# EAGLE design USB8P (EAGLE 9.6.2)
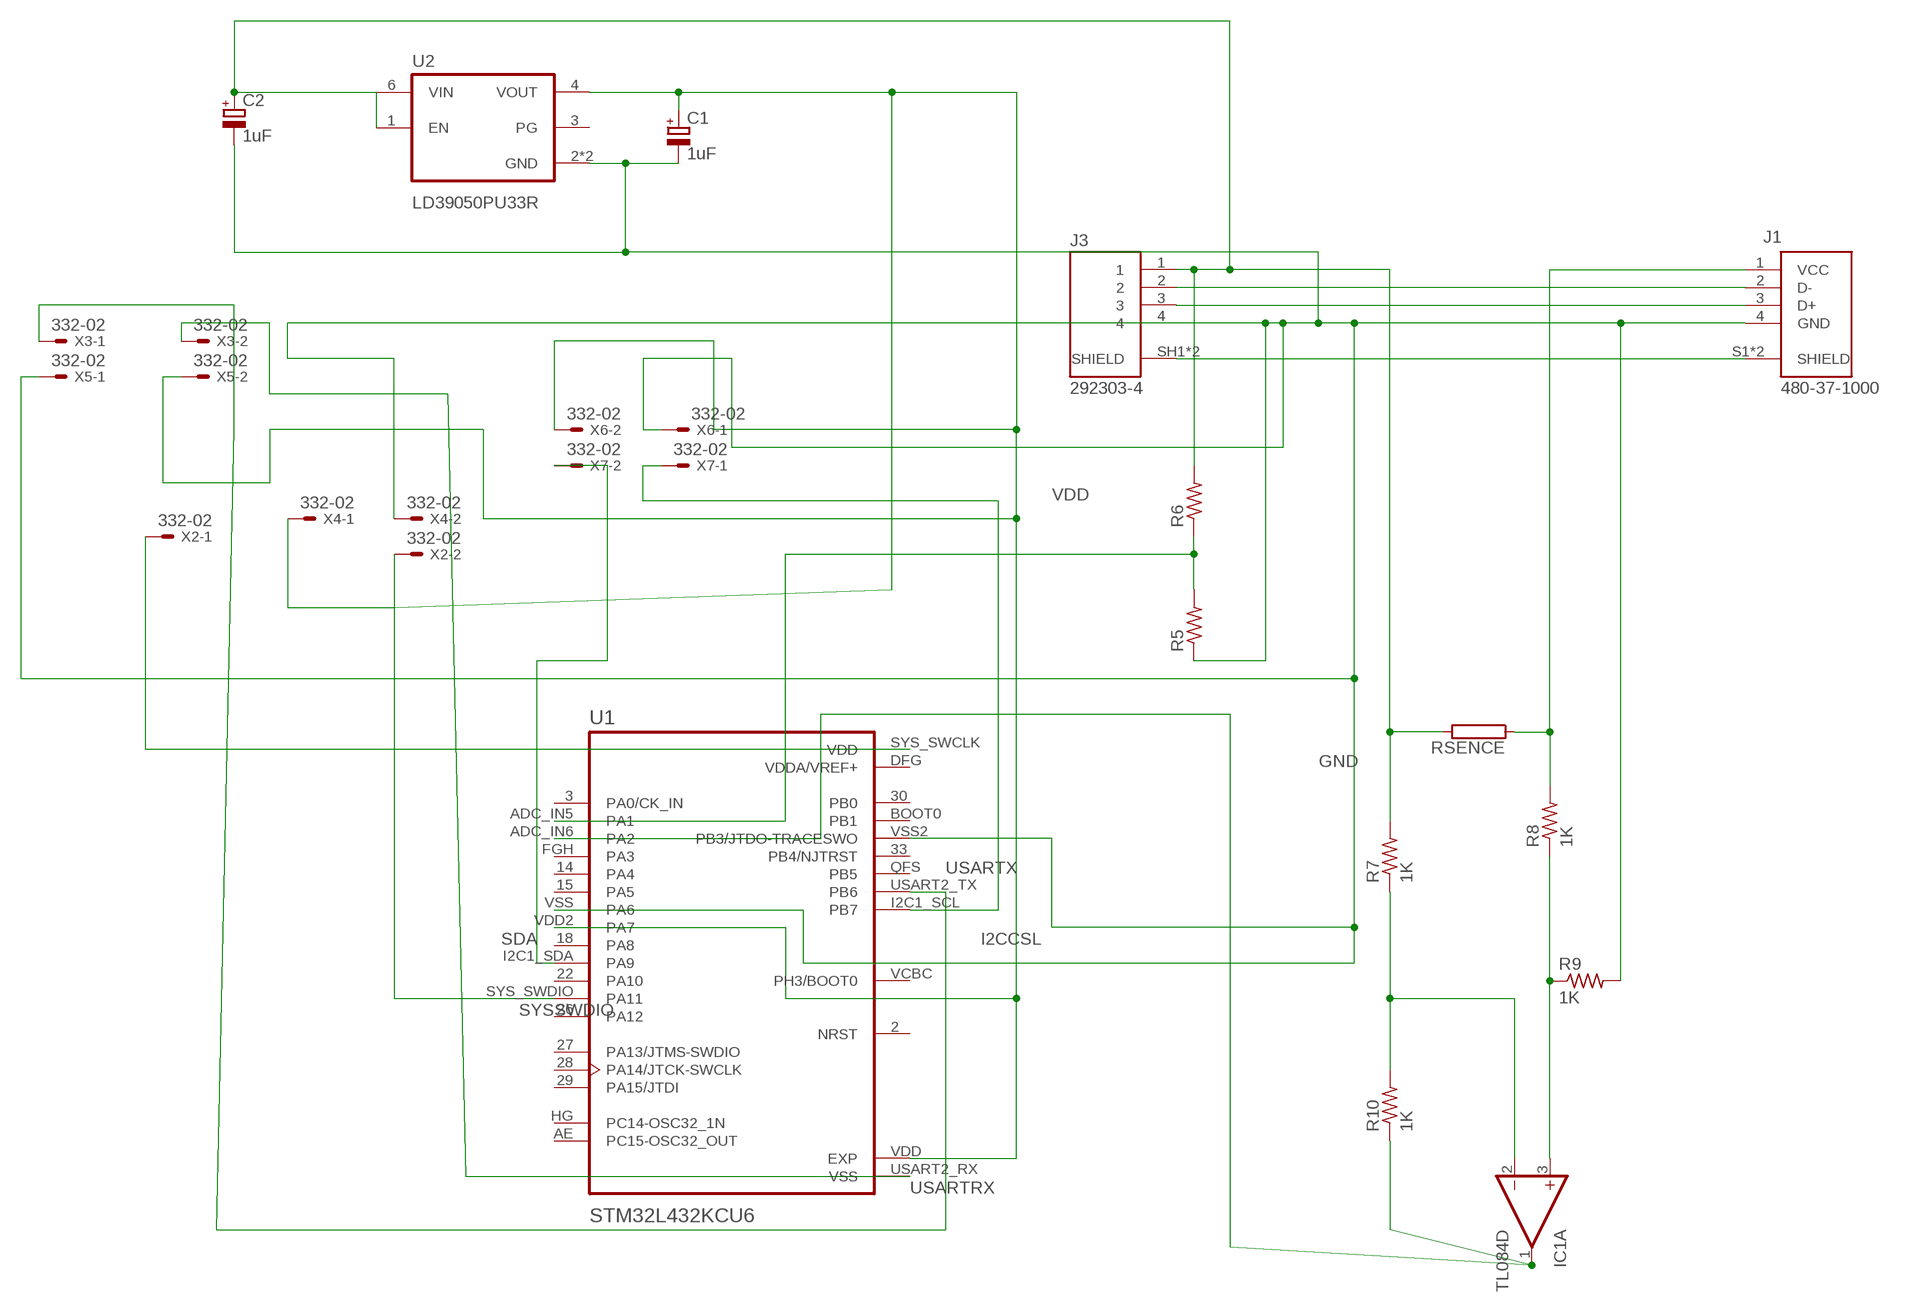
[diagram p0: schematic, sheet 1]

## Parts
C1  1uF  CPOL-EUE1.8-4  [E1,8-4]
C2  1uF  CPOL-EUE1.8-4  [E1,8-4]
IC1  TL084D  [SO14]
J1  480-37-1000  [MOLEX_480-37-1000]
J3  292303-4  [TE_292303-4]
R5  R-US_R1206  [R1206]
R6  R-US_R1206  [R1206]
R7  1K  R-US_R1206  [R1206]
R8  1K  R-US_R1206  [R1206]
R9  1K  R-US_R1206  [R1206]
R10  1K  R-US_R1206  [R1206]
RSENCE  RHPS58  [HPS58]
U1  STM32L432KCU6  [QFN50P500X500X60-33N]
U2  LD39050PU33R  [SON95P300X300X100-7N]
X2  332-02  [332-02]
X3  332-02  [332-02]
X4  332-02  [332-02]
X5  332-02  [332-02]
X6  332-02  [332-02]
X7  332-02  [332-02]

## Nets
GND: C1.- C2.- J1.4(GND) J3.4 R5.1 R9.2 U1.VSS2(PB3/JTDO-TRACESWO) U1.VSS(PA6) U2.2(GND) U2.7(GND) X4.2 X5.1 X6.1
I2CCSL: U1.I2C1_SCL(PB7) X7.1
N$1: IC1.2(A:-IN) R7.1 R10.2
N$2: IC1.3(A:+IN) R8.1 R9.1
N$3: IC1.1(A:OUT) R10.1 U1.ADC_IN6(PA2)
N$4: C2.+ J3.1 R6.2 R7.2 RSENCE.2 U2.1(EN) U2.6(VIN)
N$6: J1.2(D-) J3.2
N$7: J1.3(D+) J3.3
N$9: J1.S1(SHIELD) J1.S2(SHIELD) J3.SH1(SHIELD) J3.SH2(SHIELD)
N$10: R5.2 R6.1 U1.ADC_IN5(PA1)
N$12: U1.SYS_SWCLK(VDD) X2.1
SDA: U1.I2C1_SDA(PA9) X7.2
SYSSWDIO: U1.SYS_SWDIO(PA11) X2.2
USARTRX: U1.USART2_RX(VSS) X3.2
USARTX: U1.USART2_TX(PB6) X3.1
VCC: J1.1(VCC) R8.2 RSENCE.1
VDD: C1.+ U1.VDD2(PA7) U1.VDD(EXP) U2.4(VOUT) X4.1 X5.2 X6.2
Unconnected: IC1.5(B:+IN) IC1.6(B:-IN) IC1.7(B:OUT) IC1.8(C:OUT) IC1.9(C:-IN) IC1.10(C:+IN) IC1.12(D:+IN) IC1.13(D:-IN) IC1.14(D:OUT) U1.2(NRST) U1.3(PA0/CK_IN) U1.14(PA4) U1.15(PA5) U1.18(PA8) U1.22(PA10) U1.26(PA12) U1.27(PA13/JTMS-SWDIO) U1.28(PA14/JTCK-SWCLK) U1.29(PA15/JTDI) U1.30(PB0) U1.33(PB4/NJTRST) U1.AE(PC15-OSC32_OUT) U1.BOOT0(PB1) U1.FGH(PA3) U1.HG(PC14-OSC32_1N) U1.QFS(PB5) U1.VCBC(PH3/BOOT0) U2.3(PG)

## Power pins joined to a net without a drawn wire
GND: IC1.11(P:V-)
VCC: IC1.4(P:V+)
VDDA/VREF+: U1.DFG(VDDA/VREF+)

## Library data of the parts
C1 C2 = rcl:CPOL-EU: POLARIZED CAPACITOR, European symbol; SPICEPREFIX: C
IC1 = linear:TL084: OP AMP
J1 = 480-37-1000:480-37-1000: USB-A (USB TYPE-A) USB 2.0 Plug Connector 4 Position Surface Mount, Right Angle; Through Hole; AVAILABILITY: Unavailable; DESCRIPTION: USB-A (USB TYPE-A) USB 2.0 Plug Connector 4 Position Surface Mount, Right Angle; Through Hole; MF: Molex; MP: 480-37-1000; PACKAGE: FakePackage u; PRICE: None
J3 = 292303-4:292303-4: CONN USB TYPE A R/A PCB Check prices; AVAILABILITY: Good; COMMENT: 292303-4; DESCRIPTION: Conn; Data; USB; Recept; 2.0; 4 Pos; 1 Port; Rt Angle; A Ser; Tin over Copper; EU_ROHS_COMPLIANCE: Compliant; MF: TE Connectivity; MP: 292303-4; PACKAGE: None; PRICE: None; PURCHASE-URL: https://pricing.snapeda.com/search/part/292303-4/?ref=eda
R5-R10 = rcl:R-US_: RESISTOR, American symbol; SPICEPREFIX: R
RSENCE = resistor-power:R: Power Resitor; OC_FARNELL: unknown; OC_NEWARK: unknown
U1 = STM32G030K6:STM32L432KCU6: None Check prices; AVAILABILITY: Good; DESCRIPTION: ARM® Cortex®-M4 STM32L4 Microcontroller IC 32-Bit 80MHz 256KB (256K x 8) FLASH 32-UFQFPN (5x5); MF: STMicroelectronics; MP: STM32L432KCU6; PACKAGE: UFQFN-32 STMicroelectronics; PRICE: None; PURCHASE-URL: https://pricing.snapeda.com/search/part/STM32L432KCU6/?ref=eda
U2 = LD39050PU33R:LD39050PU33R: LD39050 Series 500 mA 3.3 V Fixed Low Noise LDO Voltage Regulator - DFN-6 Check prices; AVAILABILITY: Good; DESCRIPTION: Linear Voltage Regulator IC Positive Fixed 1 Output 500mA 6-DFN (3x3); MF: STMicroelectronics; MP: LD39050PU33R; PACKAGE: DFN-6 STMicroelectronics; PRICE: None; PURCHASE-URL: https://pricing.snapeda.com/search/part/LD39050PU33R/?ref=eda
X2-X7 = con-garry:332-02: 2 Pin - 2mm Dual Row

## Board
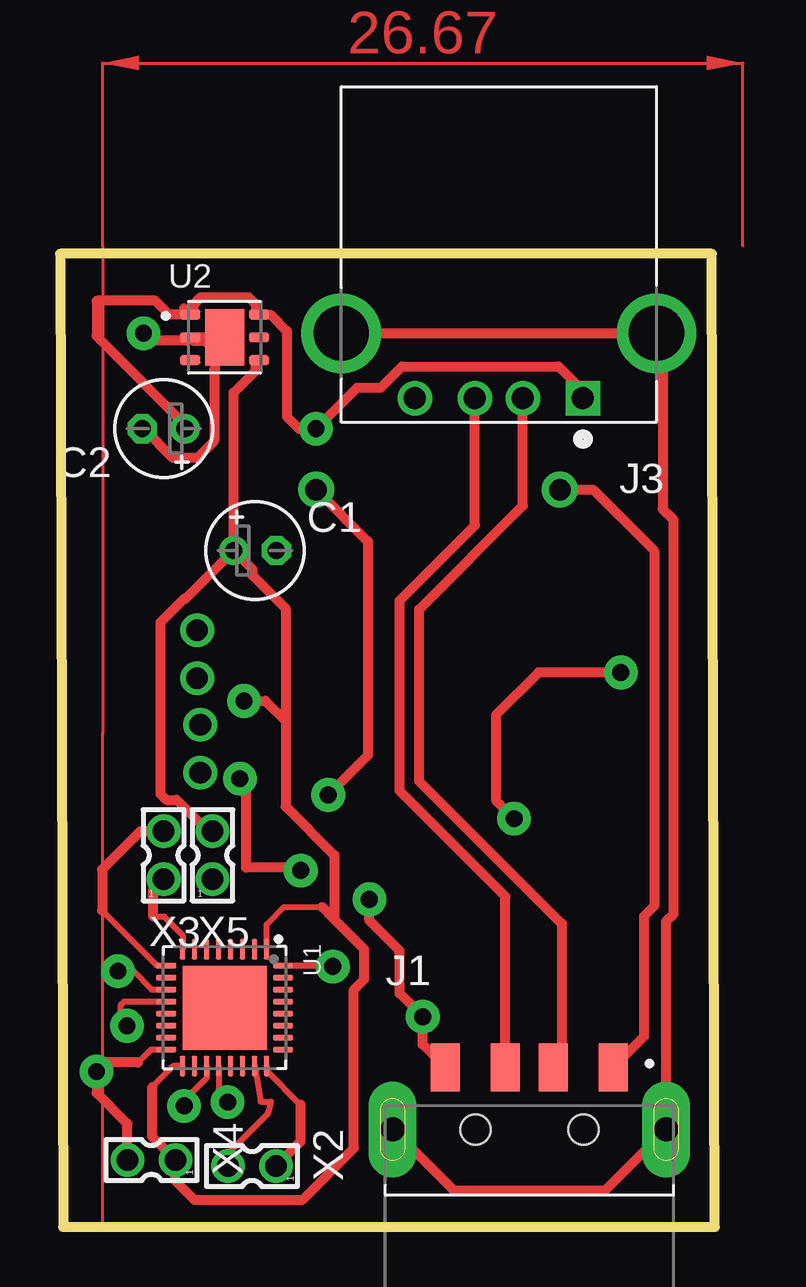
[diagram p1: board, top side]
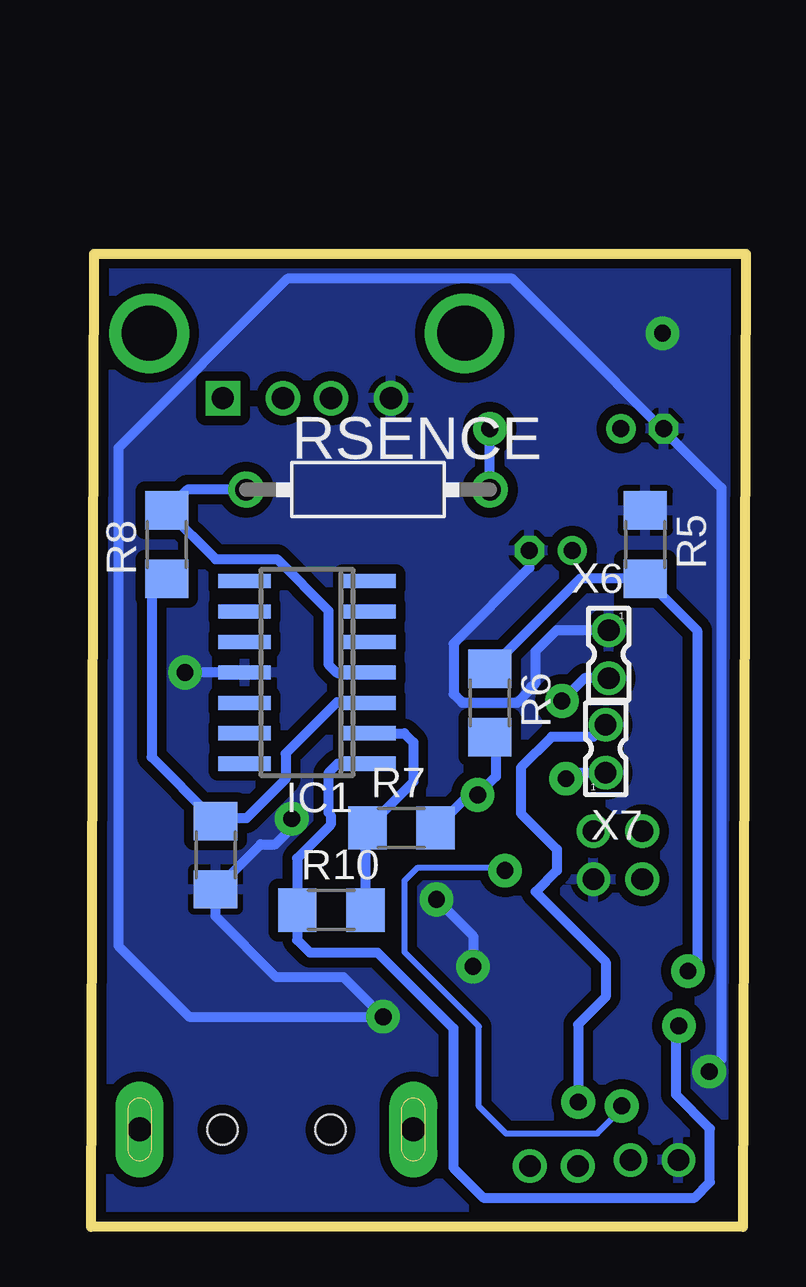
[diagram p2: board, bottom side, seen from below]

Size 27.29 x 40.56 mm. Coordinates in mm from the lower left corner, seen from the top.
Outline: 0.13,0 27.29,0 27.16,40.56 0,40.56 0.13,0
Copper layers (1*16): Top 0.035mm / dielectric 1.5mm / Bottom 0.035mm
Design rules "default *": minimum track width 16mil, minimum drill 0.35mm, track to track 16mil, track to pad 16mil, pad to pad 16mil, via to via 16mil, smd to smd 16mil, copper to edge 16mil, drill to drill 6mil, minimum pad ring 10mil, minimum via ring 8mil, stop-mask expansion 4mil, vias tented up to drill 0mil, thermal gap 10mil

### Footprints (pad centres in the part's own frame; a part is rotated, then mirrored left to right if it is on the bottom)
E1,8-4 = drill 0.711 pad 1.168: + -0.889,0 | drill 0.711 pad 1.168 octagon: - 0.889,0
SO14 = smd 0.6 x 2.2: 1 -3.81,-2.6; 2 -2.54,-2.6; 3 -1.27,-2.6; 4 0,-2.6; 5 1.27,-2.6; 6 2.54,-2.6; 7 3.81,-2.6; 8 3.81,2.6; 9 2.54,2.6; 10 1.27,2.6; 11 0,2.6; 12 -1.27,2.6; 13 -2.54,2.6; 14 -3.81,2.6
MOLEX_480-37-1000 = smd 1.2 x 2: 1 3.5,2.6; 2 1,2.6; 3 -1,2.6; 4 -3.5,2.6 | drill 1 pad 2 long: S1 -5.7,0; S2 5.7,0 | hole 1.25: -2.25,0; 2.25,0
TE_292303-4 = drill 0.92 square: 1 -3.5,0 | drill 0.92: 2 -1,0; 3 1,0; 4 3.5,0 | drill 2.3: SH1 -6.57,-2.71; SH2 6.57,-2.71
R1206 = smd 1.6 x 1.803: 1 -1.422,0; 2 1.422,0
HPS58 = drill 0.9 pad 1.5: 1 -5.08,0; 2 5.08,0
QFN50P500X500X60-33N = smd 0.86 x 0.25: 2 -2.435,1.25; 3 -2.435,0.75; 18 2.435,-1.25; 22 2.435,0.75; AE -2.435,-0.75; HG 2.435,0.25; I2C1_SCL 2.435,-0.75; I2C1_SDA 2.435,-0.25; NRST -2.435,0.25; QFS -2.435,-1.25; SYS_SWCLK 2.435,1.75; SYS_SWDIO 2.435,1.25; USART2_TX -2.435,-1.75; VDD -2.435,1.75; VDD2 2.435,-1.75; VDDA -2.435,-0.25 | smd 0.25 x 0.86: 14 0.75,-2.435; 15 1.25,-2.435; 26 1.25,2.435; 27 0.75,2.435; 28 0.25,2.435; 29 -0.25,2.435; 30 -0.75,2.435; ADC_IN5 -0.75,-2.435; ADC_IN6 -0.25,-2.435; BOOT0 -1.25,2.435; DFG -1.25,-2.435; FGH 0.25,-2.435; USART2_RX -1.75,-2.435; VCBC 1.75,2.435; VSS 1.75,-2.435; VSS2 -1.75,2.435 | smd 3.5 x 3.5: 33 0,0
SON95P300X300X100-7N = smd 0.84 x 0.4: 1 -1.435,0.95; 2 -1.435,0; 3 -1.435,-0.95; 4 1.435,-0.95; 5 1.435,0; 6 1.435,0.95 | smd 1.625 x 2.365: 7 0,0
332-02 = drill 0.9 pad 1.27: 1 0,-1; 2 0,1

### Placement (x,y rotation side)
C1  8.13,28.19 0 top
C2  4.32,33.27 180 top
IC1  18.29,23.11 90 bottom
J1  19.56,4.06 0 top
J3  18.29,34.54 180 top
R5  4.19,28.45 270 bottom
R6  10.67,21.84 270 bottom
R7  14.35,16.64 0 bottom
R8  24.13,28.45 90 bottom
R9  22.1,15.49 270 bottom
R10  17.27,13.21 0 bottom
RSENCE  15.75,30.73 0 bottom
U1  6.86,9.14 270 top
U2  6.86,37.08 0 top
X2  8,2.54 90 top
X3  4.32,15.49 0 top
X4  3.81,2.79 90 top
X5  6.35,15.49 0 top
X6  5.71,23.88 180 bottom
X7  5.84,19.94 0 bottom

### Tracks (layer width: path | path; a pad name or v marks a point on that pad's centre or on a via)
GND  (via drill 0.7 pad 1.4)
  Top 0.254: U1.VSS 3.79,7.39 3.25,6.86 | U1.VSS2 11.33,10.89 v11.37,10.86
  Top 0.406: U2.2 5.56,36.94 6.04,36.94 6.45,36.53 6.45,35.74 6.43,35.71 6.43,32.77 5.71,32.05 4.7,32.05 3.48,33.27 C2.- | U2.2 5.28,36.94 3.79,36.94 v3.48,37.25 | J1.4 15.11,7.61 v15.11,8.76 14.15,9.73 14.15,11.51 12.89,12.77 v12.89,13.65 | 3.25,6.86 1.91,6.86 v1.52,6.48 1.52,5.59 2.81,4.3 X4.2 | v11.37,10.86 11.43,10.92 | U2.2 U2.7 | v23.37,23.11 19.94,23.11 18.16,21.34 18.16,17.78 v18.92,17.02
  Bottom 0.406: v15.11,8.76 16.76,10.41 19.56,10.41 22.1,12.95 R9.2 20.22,15.95 19.6,15.95 18.92,16.63 v18.92,17.02 | v15.11,8.76 15.15,8.8 | v1.52,6.48 1.02,6.98 1.02,30.81 9.73,39.52 19.1,39.52 26.15,32.47 26.15,11.72 23.19,8.76 v15.11,8.76 | IC1.11 v23.37,23.11 | v12.89,13.65 11.37,12.13 v11.37,10.86 | C1.- 9.02,27.48 12.18,24.32 12.18,22.21 11.82,21.86 9.51,21.86 8.97,22.39 8.97,22.47 8.76,22.68 8.76,24 7.89,24.88 X6.1 6.49,24.88
  pour Bottom: 0.13,40.89 0.13,0.13 27.18,0.13 27.18,40.89
I2CCSL  (via drill 0.7 pad 1.4)
  Top 0.254: v5.17,5.04 5.17,5.28 6.11,6.21 U1.I2C1_SCL
  Top 0.406: v10.03,14.86 9.91,14.99 7.75,14.99 7.75,18.3 7.49,18.56 v7.49,18.69
  Bottom 0.254: 5.17,4.92 6.19,3.9 10,3.9 11.12,5.03 11.12,8.36 14.22,11.46 14.22,14.43 13.67,14.99 10.16,14.99
  Bottom 0.406: v7.49,18.69 7.24,18.94 X7.1 | v5.17,5.04 5.17,4.92 | 10.16,14.99 v10.03,14.86
N$1
  Bottom 0.406: 15.58,20.47 IC1.2 14.22,20.57 13.85,20.2 13.85,18.56 R7.1 15.85,16.56 R10.2
N$2
  Bottom 0.406: 24.28,27.03 R8.1 24.76,26.39 24.76,19.58 22.21,17.03 | IC1.3 15.71,21.87 17.04,21.87 19.18,19.73 19.18,18.67 20.82,17.03 22.21,17.03 | 21.95,16.76 R9.1 22.21,17.03
N$3  (via drill 0.7 pad 1.4)
  Top 0.254: U1.ADC_IN6 2.67,9.39 2.54,9.27 2.54,8.64
  Top 0.406: 2.67,8.51 v2.79,8.38 2.54,8.64
  Bottom 0.406: IC1.1 17.02,19.3 17.4,18.92 17.4,17.27 17.3,17.17 17.3,16.76 18.69,15.37 R10.1 18.69,11.96 18.16,11.43 15.34,11.43 12.19,8.28 12.19,2.48 10.94,1.23 2.14,1.23 1.5,1.87 1.5,4.1 2.92,5.53 2.92,8.25 v2.79,8.38
N$4  (via drill 0.7 pad 1.4)
  Top 0.406: U2.1 5.56,38.17 5.56,38.47 5.85,38.75 7.87,38.75 8.15,38.47 8.15,38.17 U2.6 8.31,38.02 8.78,38.02 9.45,37.35 9.45,33.77 9.95,33.27 v10.67,33.27 12.38,34.99 13.36,34.99 14.24,35.87 20.77,35.87 21.79,34.85 J3.1 | C2.+ 5.21,33.45 1.52,37.14 1.52,38.61 3.98,38.61 4.55,38.03 U2.1 | U2.1 5.17,38.29 | RSENCE.2 12.83,28.58 12.83,19.66 v11.18,18.01
  Bottom 0.406: R7.2 11.56,18.01 v11.18,18.01 10.41,18.77 10.41,20.17 R6.2 | RSENCE.2 v10.67,33.27
N$6
  Top 0.406: J3.2 19.29,30.07 14.96,25.74 14.96,18.58 20.91,12.63 20.91,7.02 J1.2
N$7
  Top 0.406: J3.3 17.29,29.24 14.15,26.1 14.15,18.18 18.56,13.78 J1.3
N$9
  Top 0.406: J3.SH2 J3.SH1 25.11,37 25.11,29.93 25.56,29.48 25.56,13.04 25.26,12.73 J1.S2 22.72,1.52 16.4,1.52 J1.S1
N$10  (via drill 0.7 pad 1.4)
  Top 0.254: U1.ADC_IN5 3.82,9.89 3.05,10.67 v2.41,10.67
  Bottom 0.406: R6.1 6.91,27.03 R5.2 2.03,24.87 2.03,11.05 v2.41,10.67
N$12
  Top 0.254: U1.SYS_SWCLK 8.61,6.51 10.02,5.1
  Top 0.406: X2.1 10.02,3.56 10.02,5.1
SDA  (via drill 0.7 pad 1.4)
  Top 0.254: v6.98,5.21 6.98,5.32 6.61,5.69 U1.I2C1_SDA
  Bottom 0.406: v6.98,5.21 6.98,8.44 5.84,9.58 5.84,11.05 8.76,13.97 7.87,14.86 7.87,15.75 9.37,17.25 9.37,19.15 8.1,20.43 6.35,20.43 X7.2
SYSSWDIO
  Top 0.254: U1.SYS_SWDIO 8.36,5.23 8.78,5.23 8.68,4.79 8.68,4.74 7,3.06
  Top 0.406: X2.2 7,3.06
USARTRX
  Top 0.254: U1.USART2_RX 4.04,10.89 1.76,13.18
  Top 0.406: 1.76,13.18 1.76,14.9 3.35,16.49 X3.2
USARTX
  Top 0.254: U1.USART2_TX 5.11,12.16 4.35,12.93 3.89,12.93
  Top 0.406: 3.89,12.93 3.89,14.06 X3.1
VCC
  Top 0.406: J1.1 24.33,7.93 24.33,12.95 24.75,13.38 24.75,28.19 22.21,30.73 RSENCE.1
  Bottom 0.406: RSENCE.1 23.27,30.73 R8.2 22.09,27.83 19.54,27.83 17.4,25.7 17.4,23.45 17.04,23.09 15.71,23.09 IC1.4
VDD  (via drill 0.7 pad 1.4)
  Top 0.254: U1.VDD2 4.73,6.71 3.85,5.84 | 10.92,13.33 9.35,13.33 8.61,12.59 U1.VDD
  Top 0.406: U2.4 8.15,35.99 8.15,35.7 7.24,34.79 C1.+ | 11.43,12.83 11.43,15.49 9.4,17.53 9.4,21.08 | 9.4,21.08 9.4,25.78 8.01,27.17 8.01,27.43 C1.+ | 3.85,5.84 3.85,3.75 X4.1 4.81,1.92 5.59,1.14 10.11,1.14 12.25,3.28 12.25,9.89 12.68,10.32 12.68,11.58 11.43,12.83 | v7.67,21.93 8.55,21.93 9.4,21.08 | X5.2 6.18,16.49 4.86,17.81 4.42,17.81 4.19,18.03 4.19,25.21 5.17,26.19 5.23,26.19 C1.+ | 11.43,12.83 10.92,13.33
  Bottom 0.406: X6.2 6.72,22.88 v7.67,21.93
(copper drawn outside any net)
  shapes: Top area x3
